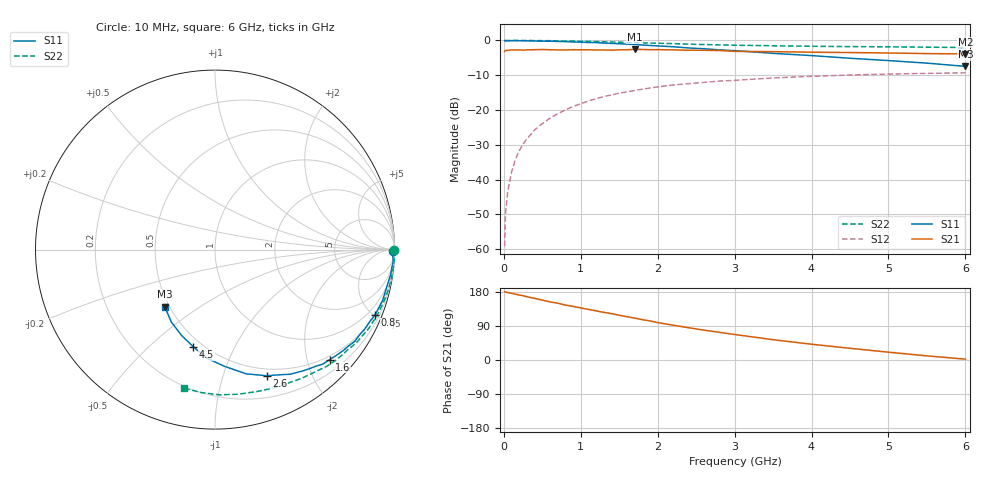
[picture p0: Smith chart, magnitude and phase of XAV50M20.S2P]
! SIEMENS Discrete & RF Semiconductors
! BFY180
! Si NPN RF Bipolar Junction Transistor in MICRO-X
! VCE = 0.5 V  IC = 0.2 mA
! Common Emitter S-Parameters:  May  1997
# GHz  S  MA  R  50
!  f  S11  S21  S12  S22
! GHz  MAG  ANG  MAG  ANG  MAG  ANG  MAG  ANG
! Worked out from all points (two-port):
!   36 points, 10 MHz to 6 GHz, reference 50 ohm
!   highest |S21| = -2.57 dB at 1.7 GHz (marker M1); lowest = -3.9 dB at 6 GHz (marker M2)
!   |S21| within 3 dB of the highest: start of sweep to end of sweep
!   lowest |S11| = -7.5 dB at 6 GHz (marker M3), VSWR 2.47, Z = 23.6 - j18.3 ohm
!   |S11| at or under -10 dB: nowhere
!   |S22| runs from -2.0 to 0.0 dB; largest |S21 - S12| = 0.73
!   S11 on the Smith chart (normalised r, x): 10 MHz: open; 800 MHz: 0.51, -5.02; 1.6 GHz: 0.43, -2.42; 2.6 GHz: 0.42, -1.40; 4.5 GHz: 0.45, -0.70; 6 GHz: 0.47, -0.37
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0.01  0.9917 -0.3  0.694 179.9  0.0011 85.6  0.9978 -0.1
0.02  0.9824 -0.6  0.717 179.2  0.0031 86.3  0.9999 -0.5
0.05  0.9872 -1.2  0.719 178.2  0.0067 89.1  0.9998 -1.1
0.1  0.9934 -2.8  0.73 176.0  0.0127 88.5  0.9971 -2.3
0.15  0.9943 -4.3  0.731 173.8  0.0194 87.0  0.9999 -3.4
0.2  0.9901 -5.6  0.731 171.4  0.0259 86.0  0.9983 -4.5
0.3  0.9879 -8.3  0.732 166.9  0.0385 82.7  0.9966 -6.7
0.4  0.981 -11.2  0.737 162.7  0.0515 80.6  0.9962 -9.0
0.6  0.9757 -16.8  0.735 153.3  0.0763 75.3  0.9908 -13.4
0.8  0.9621 -22.3  0.729 144.8  0.1 70.2  0.9819 -18.0
1.1  0.9353 -30.5  0.734 133.5  0.1343 62.8  0.968 -24.5
1.6  0.8853 -43.8  0.735 114.2  0.1826 51.2  0.9359 -35.0
1.7  0.8764 -46.7  0.744 110.8  0.1905 49.0  0.9264 -36.9
2.2  0.8116 -58.8  0.732 91.9  0.229 38.6  0.9002 -46.3
2.6  0.7596 -67.7  0.722 78.7  0.2494 31.7  0.8733 -52.9
3  0.7137 -75.9  0.697 67.3  0.2668 24.9  0.8535 -59.3
3.5  0.6527 -85.3  0.69 53.6  0.2889 18.2  0.8391 -66.5
4  0.6058 -94.4  0.677 41.6  0.3046 11.1  0.8244 -73.8
4.5  0.5545 -102.6  0.67 30.9  0.3181 4.7  0.8159 -81.0
5  0.5137 -111.2  0.66 20.6  0.3288 -1.7  0.8094 -88.2
5.5  0.4717 -121.0  0.647 10.9  0.3362 -7.8  0.8001 -95.5
6  0.4238 -131.3  0.64 2.2  0.3423 -14.2  0.7913 -102.6
